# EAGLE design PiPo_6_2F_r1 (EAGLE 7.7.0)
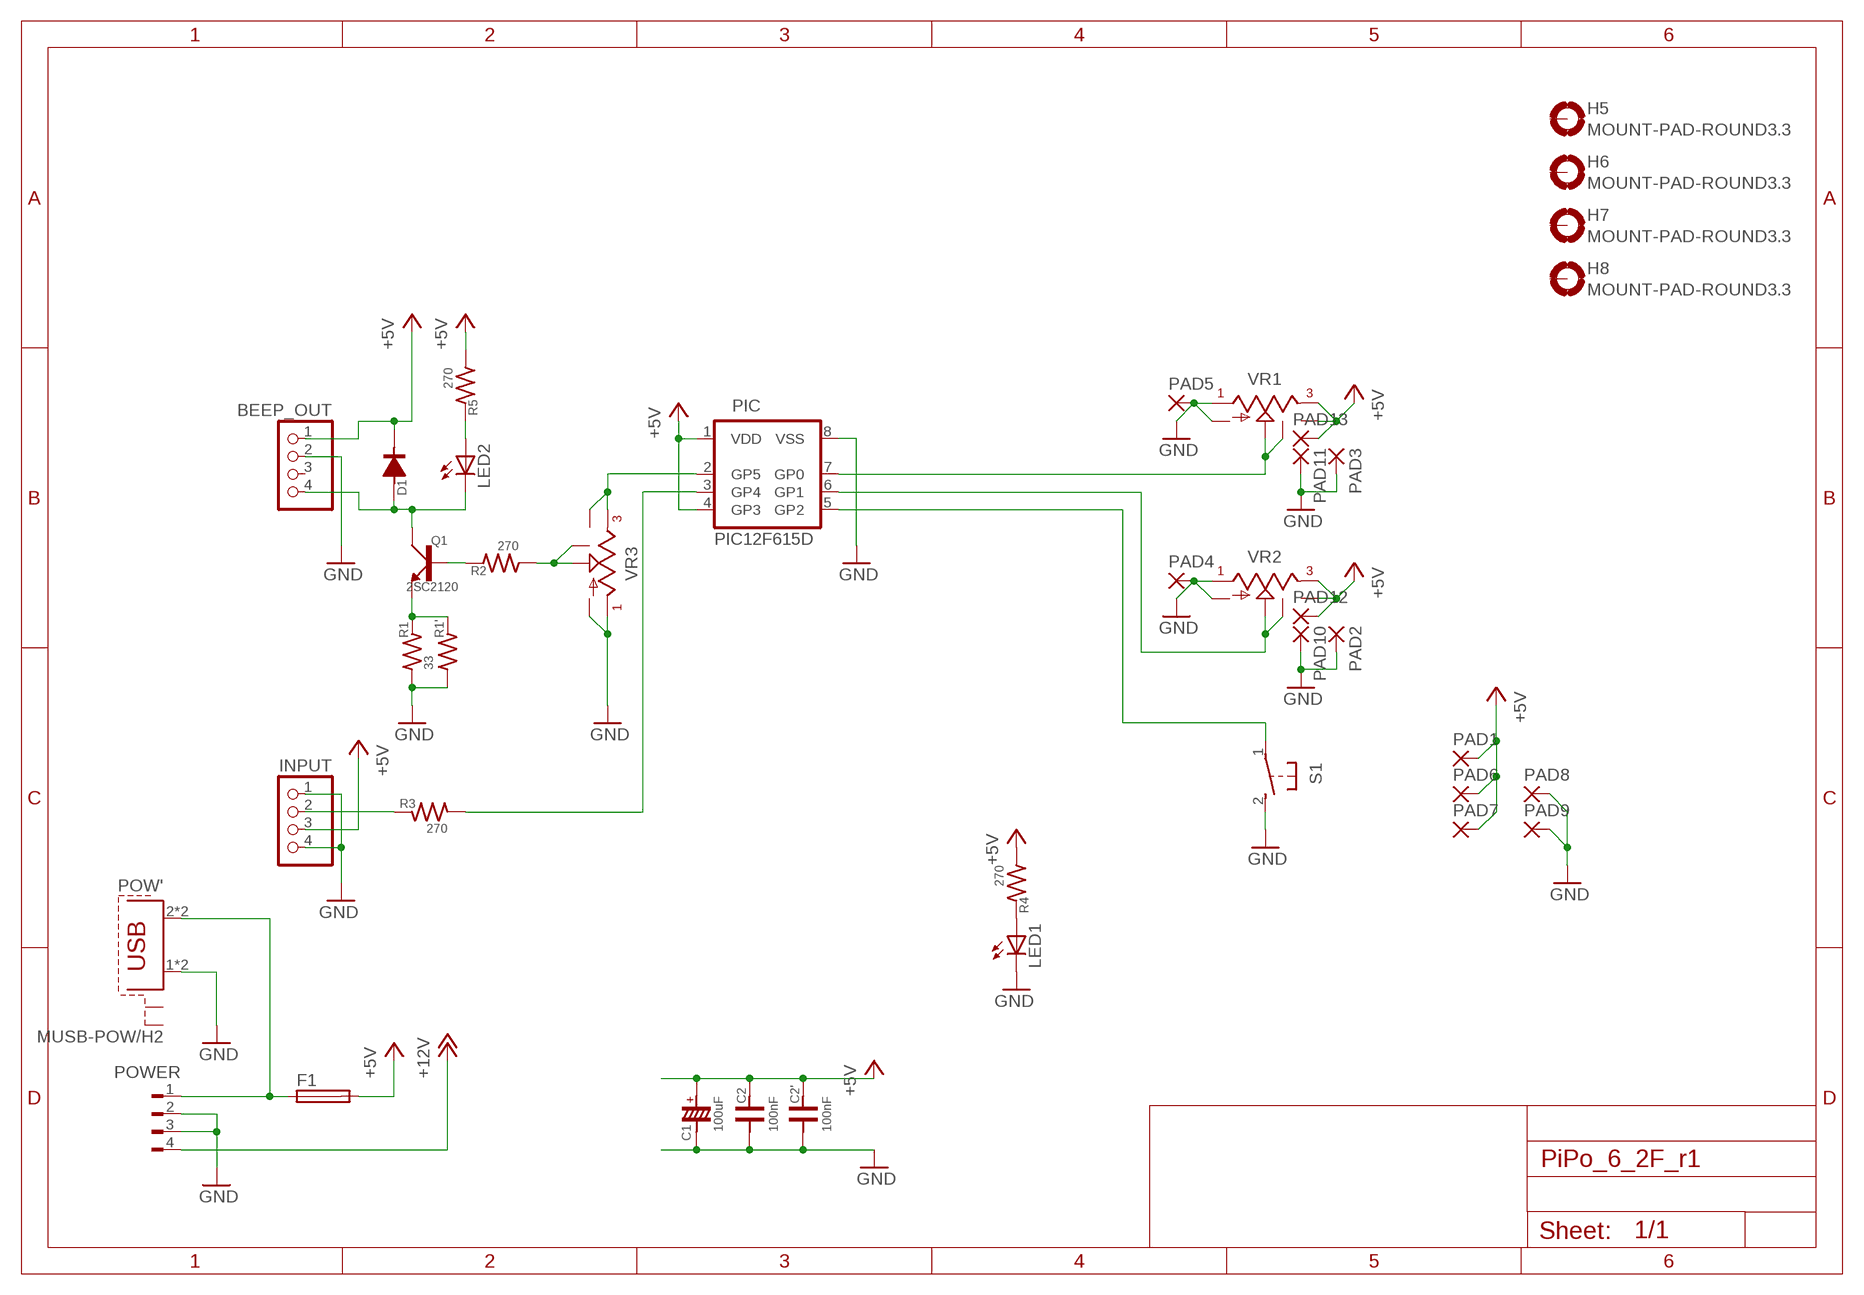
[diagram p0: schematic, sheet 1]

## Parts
BEEP_OUT  PINHD-1X4  [1X04]
C1  100uF  POLCD6.3  [TTD6.3]
C2  100nF  C50  [C50-25X044]
C2'  100nF  C2012B  [R0805B]
D1  DIODE7.5  [DIODE-D-7.5]
F1  TE5S  [TE5S]
H5  MOUNT-PAD-ROUND3.3  [3,3-PAD]
H6  MOUNT-PAD-ROUND3.3  [3,3-PAD]
H7  MOUNT-PAD-ROUND3.3  [3,3-PAD]
H8  MOUNT-PAD-ROUND3.3  [3,3-PAD]
INPUT  PINHD-1X4  [1X04]
LED1  LED3MM_  [LED3MM_]
LED2  LED3MM_  [LED3MM_]
PAD1  PAD1.80/1.0-NS  [1.80/1.0-NS]
PAD2  PAD1.80/1.0O-NS  [1.80/1.0O-NS]
PAD3  PAD1.80/1.0O-NS  [1.80/1.0O-NS]
PAD4  PAD1.80/1.0SQ-NS  [1.80/1.0SQ-NS]
PAD5  PAD1.80/1.0SQ-NS  [1.80/1.0SQ-NS]
PAD6  PAD1.80/1.0-NS  [1.80/1.0-NS]
PAD7  PAD1.80/1.0-NS  [1.80/1.0-NS]
PAD8  PAD1.80/1.0SQ-NS  [1.80/1.0SQ-NS]
PAD9  PAD1.80/1.0SQ-NS  [1.80/1.0SQ-NS]
PAD10  PAD1.80/1.0O-NS  [1.80/1.0O-NS]
PAD11  PAD1.80/1.0O-NS  [1.80/1.0O-NS]
PAD12  PAD1.80/1.0O-NS  [1.80/1.0O-NS]
PAD13  PAD1.80/1.0O-NS  [1.80/1.0O-NS]
PIC  PIC12F615D  PIC12F675DR8  [DIL08R_0.8]
POW'  MUSB-POW/H2  [MRUSB-2B/H2]
POWER  FLOP-4W71825-4  [171825-4]
Q1  2SC2120  [TO92-123]
R1  33  RR_400MIL_B  [0204-10B]
R1'  RR3225F  [M1210F]
R2  270  RR_300MIL  [0204-7.5]
R3  270  RR_300MIL  [0204-7.5]
R4  270  RR_300MIL  [0204-7.5]
R5  270  RR_300MIL  [0204-7.5]
S1  10_XX2C  [B3F-10_2C]
VR1  POT_UNIV  POT_UNIVMMP  [POT_UNIV_MM_PITCH]
VR2  POT_UNIV  POT_UNIVMMP  [POT_UNIV_MM_PITCH]
VR3  POT_UNIV  POT_UNIVMMP  [POT_UNIV_MM_PITCH]

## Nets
+5V: BEEP_OUT.1 C1.P$1 C2'.2 C2.2 D1.P$1 F1.2 INPUT.3 PAD1.1(P) PAD6.1(P) PAD7.1(P) PAD12.1(P) PAD13.1(P) PIC.1(VDD) PIC.4(GP3) R4.1 R5.1 VR1.E VR1.E2 VR2.E VR2.E2
+12V: POWER.4
GND: BEEP_OUT.2 C1.P$2 C2'.1 C2.1 INPUT.1 INPUT.4 LED1.K(C) PAD2.1(P) PAD3.1(P) PAD4.1(P) PAD5.1(P) PAD8.1(P) PAD9.1(P) PAD10.1(P) PAD11.1(P) PIC.8(VSS) POW'.1 POW'.1' POWER.2 POWER.3 R1'.1 R1.1 S1.2(S) VR1.A VR1.A2 VR2.A VR2.A2 VR3.A VR3.A2
N$1: PIC.6(GP1) VR2.S VR2.S2
N$2: PIC.7(GP0) VR1.S VR1.S2
N$3: PIC.2(GP5) VR3.E VR3.E2
N$4: PIC.5(GP2) S1.1(P)
N$5: PIC.3(GP4) R3.1
N$6: BEEP_OUT.4 D1.P$2 LED2.K(C) Q1.C
N$7: Q1.B R2.2
N$8: INPUT.2 R3.2
N$9: Q1.E R1'.2 R1.2
N$10: R2.1 VR3.S VR3.S2
N$12: LED1.A R4.2
N$13: LED2.A R5.2
VIN: F1.1 POW'.2 POW'.2' POWER.1
Unconnected: BEEP_OUT.3 H5.B3,3(MOUNT) H6.B3,3(MOUNT) H7.B3,3(MOUNT) H8.B3,3(MOUNT) POW'.S1 POW'.S2

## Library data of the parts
BEEP_OUT INPUT = pinhead:PINHD-1X4: PIN HEADER
C1 = jikken:POLC
C2 = my-C:C
C2' = jikken:C
D1 = jikken:DIODE
F1 = akizuki:TE5: FUSE
H5-H8 = my-holes:MOUNT-PAD-ROUND: MOUNTING PAD, round
LED1 LED2 = my-led_base:LED: LED
PAD1-PAD13 = jikken:PAD: THROUGH-HOLE PAD
PIC = jikken:PIC12F675
POW' = akizuki:MUSB-POW
POWER = MyLib:FLOP-4W: MATE N-LOCK Floppy / HDD conector Distributor: Bürklin 71F972
Q1 = jikken:2SC
R1 R1' R2-R5 = My-R:R
S1 = switch-omron:10_XX2
VR1-VR3 = VR:POT_UNIV

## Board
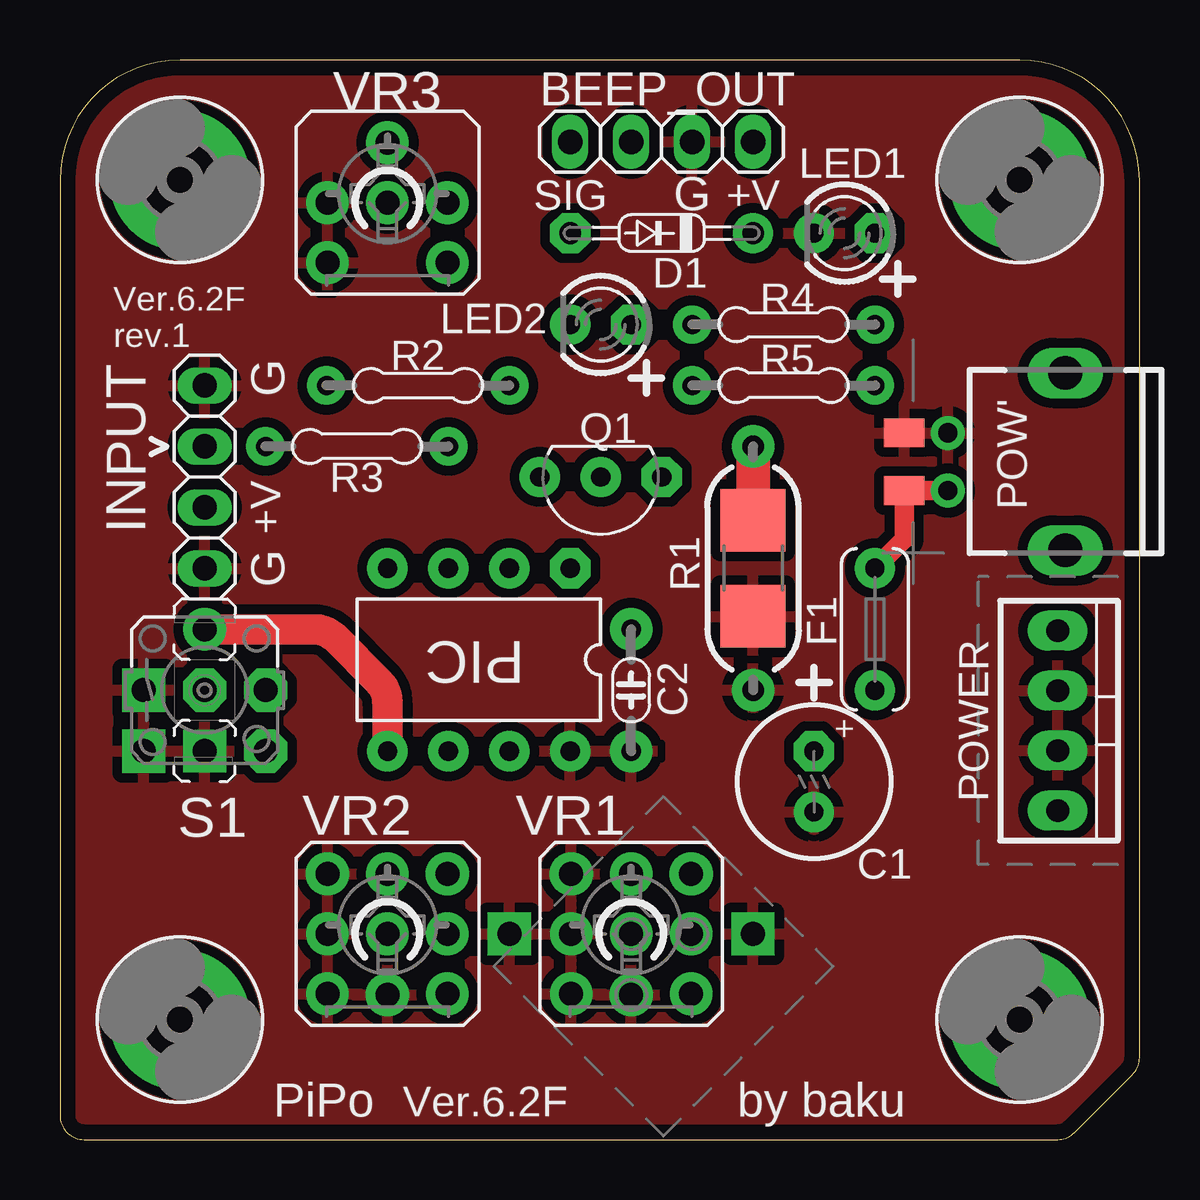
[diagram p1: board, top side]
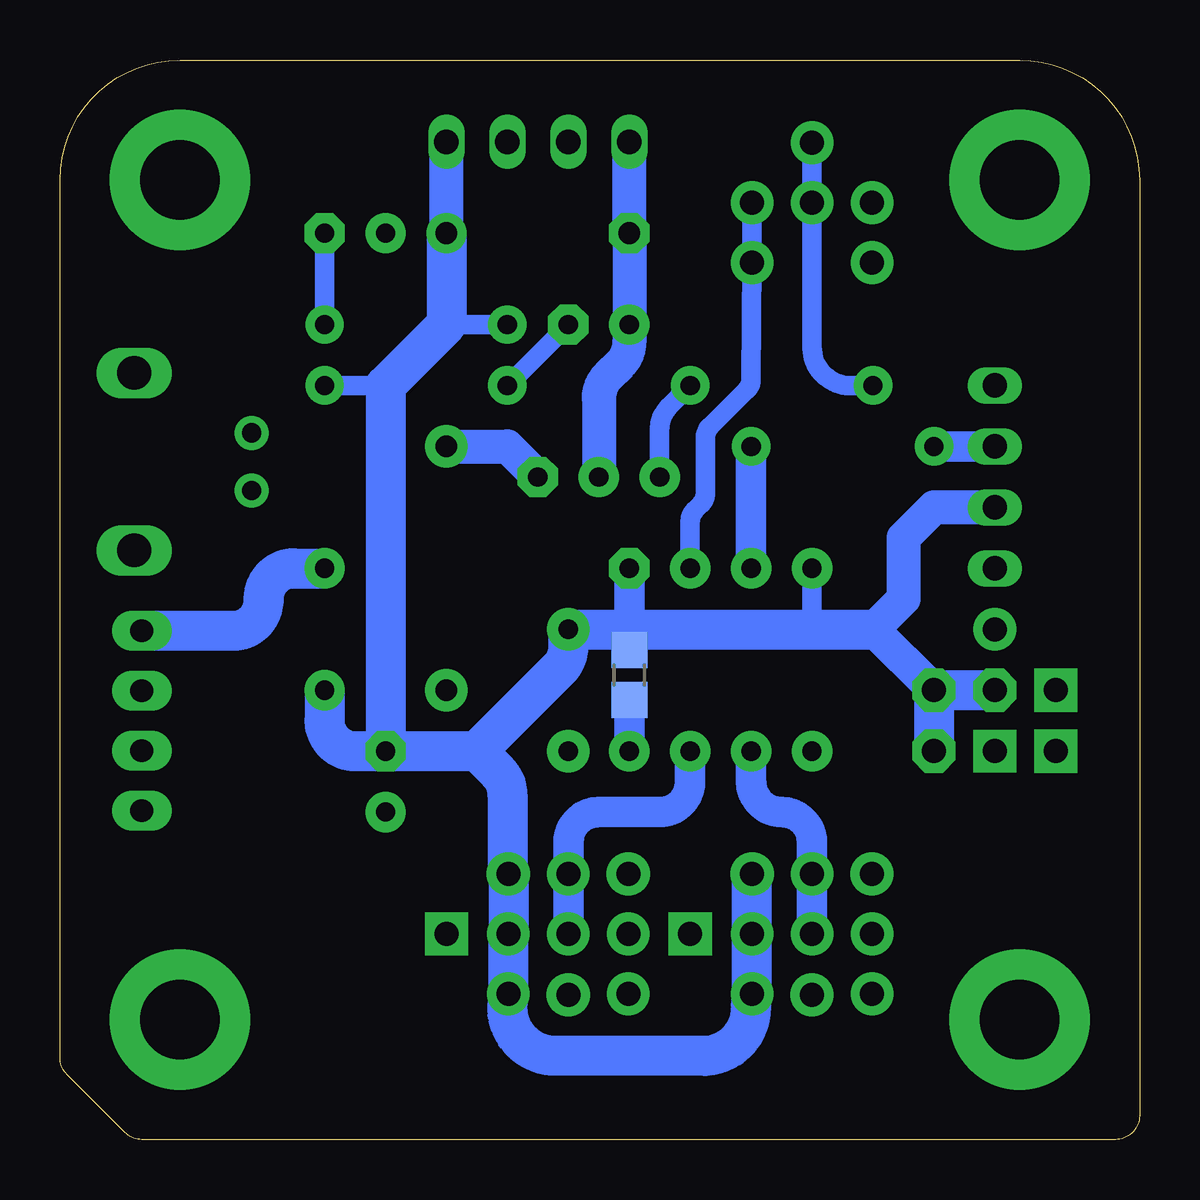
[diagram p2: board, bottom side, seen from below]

Size 45 x 45 mm. Coordinates in mm from the lower left corner, seen from the top.
Outline: 0,40 0,1 arc90 1,0 41.59,0 arc45 42.29,0.29 44.71,2.71 arc45 45,3.41 45,40 arc90 40,45 5,45 arc90 0,40
Copper layers (1*16): Top 0.035mm / dielectric 1.5mm / Bottom 0.035mm
Design rules "16mil_PiPo62A_tite *": minimum track width 10mil, minimum drill 20mil, track to track 16mil, track to pad 16mil, pad to pad 10mil, via to via 10mil, smd to smd 8mil, copper to edge 25mil, drill to drill 8mil, minimum pad ring 10mil, minimum via ring 8mil, stop-mask expansion 4mil, vias tented up to drill 0mil, thermal gap 16mil
tRestrict: 7 lines

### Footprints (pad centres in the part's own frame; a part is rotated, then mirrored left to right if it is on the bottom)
1X04 = drill 1.016 long: 1 -3.81,0; 2 -1.27,0; 3 1.27,0; 4 3.81,0
TTD6.3 = drill 0.8 pad 1.676 octagon: P$1 -1.27,0 | drill 0.8 pad 1.676: P$2 1.27,0
C50-25X044 = drill 0.8 pad 1.778: 1 -2.54,0; 2 2.54,0
R0805B = smd 1.5 x 1.5: 1 -1.05,0; 2 1.05,0
DIODE-D-7.5 = drill 0.9 pad 1.676: P$1 -3.81,0 | drill 0.9 pad 1.676 octagon: P$2 3.81,0
TE5S = drill 0.8 pad 1.676: 1 -2.54,0; 2 2.54,0
3,3-PAD = drill 3.3 pad 5.842: B3,3 0,0
LED3MM_ = drill 0.8 pad 1.676 octagon: A -1.27,0 | drill 0.8 pad 1.676: K 1.27,0
1.80/1.0-NS = drill 1 pad 1.8 octagon: 1 0,0
1.80/1.0O-NS = drill 1 pad 1.8: 1 0,0
1.80/1.0SQ-NS = drill 1 pad 1.8 square: 1 0,0
DIL08R_0.8 = drill 0.8 pad 1.676 octagon: 1 -3.81,-3.81 | drill 0.8 pad 1.676: 2 -1.27,-3.81; 3 1.27,-3.81; 4 3.81,-3.81; 5 3.81,3.81; 6 1.27,3.81; 7 -1.27,3.81; 8 -3.81,3.81
MRUSB-2B/H2 = smd 1.2 x 1.7: 1 -1.2,-6.72; 2 1.2,-6.72 | drill 0.8 pad 1.422: 1' -1.2,-4.9; 2' 1.2,-4.9 | drill 1.4 long: S1 3.7,0; S2 -3.7,0
171825-4 = drill 0.95 pad 1.676 long: 1 -3.75,0; 2 -1.25,0; 3 1.25,0; 4 3.75,0
TO92-123 = drill 0.8 pad 1.676: B 2.54,0; C 0,0 | drill 0.8 pad 1.676 octagon: E -2.54,0
0204-10B = drill 0.9 pad 1.778: 1 -5.08,0; 2 5.08,0
M1210F = smd 2.6 x 2.7: 1 -2,0; 2 2,0
0204-7.5 = drill 0.8 pad 1.6: 1 -3.81,0; 2 3.81,0
B3F-10_2C = drill 1 pad 1.778: 1 0,2.54 | drill 1 pad 1.778 square: 2 0,-2.54
POT_UNIV_MM_PITCH = drill 1 pad 1.778: A -2.5,0; A2 -2.5,-2.5; E 2.5,0; E2 2.5,-2.5; S 0,2.5; S2 0,0

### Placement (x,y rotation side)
BEEP_OUT  25.08,41.59 180 top
C1  31.43,14.92 270 top
C2  23.81,18.73 90 top
C2'  21.27,19.36 90 bottom
D1  25.08,37.78 180 top
F1  33.97,21.27 270 top
H5  5,5 90 top
H6  40,5 90 top
H7  40,40 90 top
H8  5,40 90 top
INPUT  6.03,27.62 270 top
LED1  32.7,37.78 180 top
LED2  22.54,33.97 180 top
PAD1  6.03,18.73 0 top
PAD2  11.15,11.07 0 top
PAD3  21.31,11.07 0 top
PAD4  18.73,8.57 0 top
PAD5  28.89,8.57 0 top
PAD6  8.57,16.19 180 top
PAD7  8.57,18.73 180 top
PAD8  3.49,16.19 180 top
PAD9  3.49,18.73 180 top
PAD10  13.65,6.03 0 top
PAD11  23.81,6.03 0 top
PAD12  16.15,11.07 0 top
PAD13  26.31,11.07 0 top
PIC  17.46,20 180 top
POW'  41.91,28.25 270 top
POWER  41.59,17.46 270 top
Q1  22.54,27.62 180 top
R1  28.89,23.81 90 top
R1'  28.89,23.81 90 top
R2  14.92,31.43 0 top
R3  12.38,28.89 180 top
R4  30.16,33.97 0 top
R5  30.16,31.43 180 top
S1  6.03,18.73 0 top
U$1  [3386K_DUMMY]  23.81,8.57 45 top
VR1  23.81,8.57 0 top
VR2  13.65,8.57 0 top
VR3  13.65,39.05 0 top

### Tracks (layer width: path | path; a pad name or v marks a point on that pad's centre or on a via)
+5V
  Bottom 0.813: 13.65,21.27 PIC.4 | R5.1 31.43,31.43 | R4.1 28.89,33.97
  Bottom 1.016: 21.27,21.27 C2'.2
  Bottom 1.27: 21.27,21.27 PIC.1
  Bottom 1.422: D1.P$1 BEEP_OUT.1 | INPUT.3 8.57,26.35 9.84,25.08 9.84,22.54 11.11,21.27 PAD7.1
  Bottom 1.676: PAD1.1 PAD7.1 PAD6.1 | 11.11,21.27 13.65,21.27 21.27,21.27 C2.2 23.81,20.53 arc45 24.18,19.63 27.62,16.19 | 27.62,16.19 26.72,15.29 arc45 26.35,14.39 26.35,11.11 PAD13.1 VR1.E VR1.E2 26.35,5.49 arc-90 24.35,3.49 18.19,3.49 arc-90 16.19,5.49 VR2.E2 VR2.E PAD12.1 | C1.P$1 27.62,16.19 | D1.P$1 28.89,33.97 31.43,31.43 C1.P$1 | F1.2 33.97,17.46 arc-90 32.7,16.19 C1.P$1
GND
  Bottom 1.27: PIC.8 C2'.1
  pour Top: 0,0 45,0 45,45 0,45
N$1
  Bottom 1.27: VR2.S2 VR2.S 13.65,12.38 arc-90 14.92,13.65 arc90 16.19,14.92 PIC.6
N$2
  Bottom 1.27: VR1.S2 VR1.S 23.81,12.38 arc90 22.54,13.65 20,13.65 arc-90 18.73,14.92 PIC.7
N$3
  Bottom 0.813: VR3.E VR3.E2 16.19,31.69 arc45 16.38,31.24 17.91,29.71 arc-45 18.09,29.26 18.09,26.93 arc45 18.28,26.48 18.54,26.22 arc-45 18.73,25.77 PIC.2
N$4
  Top 1.27: PIC.5 13.65,18.2 arc45 13.28,19.1 11.48,20.9 arc45 10.58,21.27 S1.1
N$5
  Bottom 1.27: PIC.3 R3.1
N$6
  Bottom 1.422: BEEP_OUT.4 D1.P$2 LED2.K 21.27,33.23 arc45 21.64,32.33 22.17,31.8 arc-45 22.54,30.9 Q1.C
N$7
  Bottom 0.813: Q1.B 20,29.63 arc45 19.63,30.53 R2.2
N$8
  Bottom 1.27: INPUT.2 R3.2
N$9
  Top 1.422: R1.2 R1'.2
  Bottom 1.422: R1.2 26.35,28.89 Q1.E
N$10
  Bottom 0.813: VR3.S VR3.S2 13.65,33.02 arc-90 12.06,31.43 R2.1
N$12
  Bottom 0.813: R4.2 LED1.A
N$13
  Bottom 0.813: LED2.A R5.2
VIN
  Top 0.813: F1.1 35.19,25.03 POW'.2 POW'.2'
  Bottom 1.676: POWER.1 37.78,21.21 arc-90 36.51,22.48 36.51,22.54 arc90 35.24,23.81 F1.1

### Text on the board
tPlace: SIG | G | +V | Ver.6.2F / rev.1 | G | +V | G | PiPo | Ver.6.2F | by baku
